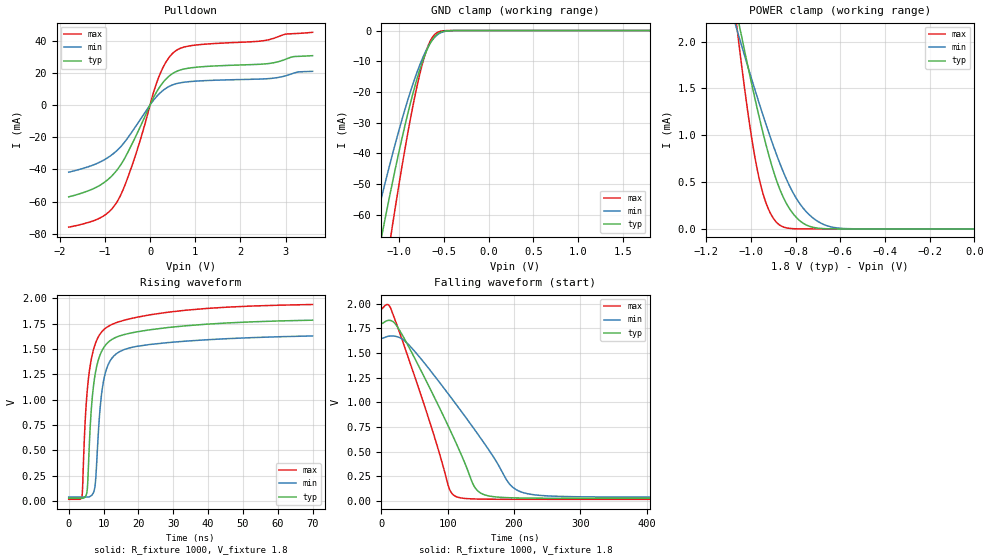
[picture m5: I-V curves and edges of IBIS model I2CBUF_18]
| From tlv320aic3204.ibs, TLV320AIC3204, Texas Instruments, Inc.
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[Model]   I2CBUF_18
Model_type  I/O_open_drain
Polarity   Inverting
Vinl=0.495
Vinh=1.365
Enable   Active-Low
Vref =   0
Rref =   1000
Cref =   10p
Vmeas =   0.9
| variable   typ   min   max
C_comp   1.40pF   1.26pF   1.49pF
| C_pulldown   1.28pF   0.05pF   3.46pF
| C_tri-state   1.40pF   1.26pF   1.49pF
[Temperature Range]   40   100   -40
| Ambient temperature   25   85   -40
[Voltage range]   1.8   1.65   1.95
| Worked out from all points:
|   slope of the pulldown table from 0 to 0.27 V, typ, clamps not added: 20.2 ohm
|   GND clamp passes 1 mA (typ) near -0.56 V on its own axis
|   POWER clamp passes 1 mA (typ) near -0.94 V on its own axis
|   rising waveform, R_fixture 1000, V_fixture 1.8: 20-80 % time 3.21ns typ, 2.94ns min, 3.42ns max; typ from 0.028 V to 1.78 V
|   falling waveform, R_fixture 1000, V_fixture 1.8: 20-80 % time 75.6ns typ, 103ns min, 56ns max; typ from 1.8 V to 0.028 V
[GND Clamp]
| I2CBUF_18
|   Voltage   I(typ)   I(min)   I(max)
-1.8V     -166.6mA   -133.3mA   -213.7mA
-1.285V   -80.68mA   -64.94mA   -104.5mA
-1.18V    -64.62mA   -52.26mA   -83.56mA
-1.08V    -50.09mA   -40.81mA   -64.32mA
-925mV    -29.6mA    -24.63mA   -36.82mA
-785mV    -14.2mA    -12.36mA   -16.1mA
-730mV    -9.343mA   -8.42mA    -9.735mA
-675mV    -5.417mA   -5.168mA   -4.874mA
-625mV    -2.826mA   -2.929mA   -2.046mA
-575mV    -1.221mA   -1.432mA   -655.8uA
-390mV    -13.01uA   -31.84uA   -1.352uA
1.8V      63.56pA    625.1pA    33.96pA
[POWER Clamp]
| I2CBUF_18
|   Voltage   I(typ)   I(min)   I(max)
-1.8V     11.83mA    8.628mA    19.35mA
-1.065V   2.333mA    2.152mA    2.209mA
-1.055V   2.216mA    2.07mA     2.012mA
-1.045V   2.1mA      1.989mA    1.819mA
-1V       1.591mA    1.63mA     1.031mA
-960mV    1.169mA    1.323mA    510.8uA
-915mV    749uA      995.8uA    180.4uA
-860mV    365.8uA    639.8uA    27.05uA
-815mV    175.7uA    404.5uA    3.749uA
-775mV    76.29uA    250.6uA    597.6nA
-655mV    1.92uA     31.22uA    2.386nA
-16.28fV  63.56pA    587.5pA    38.55pA
[Pulldown]
| I2CBUF_18
|   Voltage   I(typ)   I(min)   I(max)
-1.8V     -57.04mA   -41.72mA   -75.87mA
-1.095V   -49.62mA   -35.25mA   -70mA
-725mV    -40.15mA   -28.08mA   -59.88mA
-570mV    -33.49mA   -23.29mA   -50.77mA
-355mV    -21.72mA   -14.83mA   -34.03mA
180mV     9.744mA    6.305mA    16.35mA
355mV     16.17mA    10.43mA    26.75mA
545mV     20.32mA    12.97mA    33.2mA
940mV     23.24mA    14.7mA     37.02mA
2.655V    25.88mA    16.48mA    40.75mA
3.01V     28.54mA    18.24mA    44.09mA
3.6V      30.67mA    20.94mA    45.18mA
[Ramp]
| I2CBUF_18
| variable   typ   min   max
dV/dt_r   1.05/3.20E-09   0.95/2.94E-09   1.15/3.42E-09
dV/dt_f   1.08/7.71E-08   0.98/1.05E-07   1.18/5.73E-08
R_load = 1000
[Rising Waveform]
| I2CBUF_18
R_fixture =   1000
C_fixture =   0
L_fixture =   0
V_fixture =   1.8
V_fixture_min = 1.65
V_fixture_max = 1.95
|   Time   V(typ)   V(min)   V(max)
0s        28.4mV     40.38mV    17.94mV
3.8ns     28.22mV    40.37mV    48.67mV
5.155ns   76.95mV    40.29mV    1.021V
6.36ns    843.3mV    51.26mV    1.377V
7.27ns    1.179V     100.4mV    1.514V
7.745ns   1.282V     220.7mV    1.562V
9.105ns   1.451V     952mV      1.653V
10.48ns   1.536V     1.261V     1.703V
19.41ns   1.669V     1.526V     1.813V
70ns      1.785V     1.629V     1.939V
[Falling Waveform]
| I2CBUF_18
R_fixture =   1000
C_fixture =   0
L_fixture =   0
V_fixture =   1.8
V_fixture_min = 1.65
V_fixture_max = 1.95
|   Time   V(typ)   V(min)   V(max)
0s        1.8V       1.65V      1.95V
9.37ns    1.829V     1.668V     1.991V
14.9ns    1.828V     1.673V     1.94V
41.03ns   1.566V     1.585V     1.445V
101.8ns   746.7mV    1.078V     137.7mV
112.3ns   593mV      983.5mV    46.92mV
146.7ns   95.61mV    666.5mV    20.62mV
192.4ns   34.36mV    179.6mV    18.25mV
215.2ns   31mV       83.1mV     18.05mV
620ns     28.4mV     40.38mV    17.94mV
